| Texas Instruments Incorporated
| USB 3.0 TRANSCEIVER
| Marketing part#   Voltage Range   Package-type   Temperature
| TUSB1310IZAYR   2.97V - 3.465V   175 Ball NFBGA(175ZAY) -40C to 105C
| TUSB1310ZAY   2.97V - 3.465V   175 Ball NFBGA(175ZAY) -40C to 105C
| TUSB1310ZAYR   2.97V - 3.465V   175 Ball NFBGA(175ZAY) -40C to 105C
[IBIS Ver]   4.0
[File name]   tusb1310.ibs
[File Rev]   1.2
[Date]   05/06/2011
[Source]   Model built from TISPICE simulations at:
   Texas Instruments Incorporated.
   Analog-eLab, HPA
   12500 TI Blvd
   Dallas, TX -75243
   For Support e-mail: elab_scm_ibis@list.ti.com
[Notes]
   Rev 1.0: 06/04/2010
   - Initial version of model based on simulations from TISPICED
   - IBIS file covers only USB2.0 DP/DM and USB3.0 SSTXP/SSTXN pins only
   - For USB2.0, models are included for HS, FS and LS modes
   - For USB3.0, models are included for SATA1, SATA2 and No-De-Emphasis
   modes
   - Models are not matched to silicon or TISPICE.
   - Some of the POWER or GND balls are connected via the same net on
   package. Such ball names are commented out in the [Pin] section.
   For example, for pin B14, use the parastics of L12.
   - Warnings related to ccomp can be ignored. These reflect PVT conditions.
   Min ccomp corresponds PVT conditions related to Min. Max ccomp corresponds
   to PVT conditions related to Max
   - GND Clamp related warnings can be ignored as these reflect HS internal
   termination
   - Warnings related to USB2 LS pullup can be ignored as these are from
   simulations.
   Rev 1.1: 09/14/2010
   - Added model for DeEmphasis mode
   - Please use [Package Model] for system analysis
   - Removed parasitics from [Pin] for POWER and GND pins
   as they do not accurately represent pwr pkg parasitics
   [Package Model] includes mutuals and selfs more appropriately
   - C_comp although listed in numerical order of value are obtained from varying
   PVT conditions. For PVT conditions for each specific value refer the buffer
   description under respective [Model]. IBIS model user is responsible for using
   appropriate C_comp to simulate for Signal Integrity
   Where for TUSB1310,
   Nom PVT:  Nominal process, Typ Temperature, Typ Voltage
   Slow PVT: Weak process, Max Temperature, Min Voltage
   Fast PVT: Strong process, Min Temperatire, Max Voltage
   - ignore warning are related to usb3_WODE, please do not correct this error
   as IBIS parser does not correct IV-VT mismatch with single set of V-T
   waveforms.
   - non-monotonic arnings related to usb2_LS_RC and usb2_LS_R buffers are
   as they are seen in TISPICE simualations
   - [Driver Schedule] is interpreted differently by each system level simulator
   differently, if usual setup with it does not give appropriate results, please
   tie the MAIN and BOOST buffers as per buffer timing description under
   [Driver Schedule] keyword. For example, using HSPICE, refer DE_hspice.sp
   - Added USB High speed differential receiver model for SSRXP and SSRXN
   - Updated [Diff Pin] section.
   - Updated [Pin Mapping] section
   - Updated all USB2 model type to I/O and added Vinl and Vinh parameters
   - To test USB2 IBIS models using HSPICE look for spice set up files
   inside the TUSB1310 Correlation report
   Rev 1.2: 05/06/2011
   - [Driver Schedule] timing statements modified as per IBIS v5.0 spec.
   - Boost stage timing is set for a frequency of 1250MHz.
   - Depending on the speed grade( for various models, gen1/gen2/usb3.0 etc),
   user needs to alter the BOOST timing numbers for rise_off_dly and fall_off_dly
   usb3_de_BOOST   NA   0.2ns   NA   0.2ns
   This delay 0.2ns is valid for 1250MHz,(0.8ns period).
   Depending on the frequency, period divided by 4 needs to be used in
   DriverSchedule for BOOST
   -Ccomp interpretation needs to be assessed for accurate results. Ccomp that
   is assocaited with usb3_DE_MAIN is the complete number that includes ccomp for
   both BOOST and MAIN. Since MAIN buffer is on at all times and it is the boost
   that is turned on or ff, please set ccomp to suit your simulator's interpretation of
   IBIS v5.0 spec.
[Disclaimer] This product is designed as an aid for customers of Texas Instruments.
   No warranties, either expressed or implied, with respect to this third
   party software (if any) or with respect to its fitness for any
   particular purpose is claimed by Texas Instruments or the author. The
   software (if any) is provided solely on an "as is" basis. The entire
   risk as to its quality and performance is with the customer
[Copyright]   (C)Copyright 2010 Texas Instruments Incorporated.
   All rights reserved.
[Component]   TUSB1310
[Manufacturer]  Texas Instruments Incorporated
[Package]   |175-Ball NFBGA - ZAY package
|   typ   min   max
R_pkg   0.163   0.088   0.252
L_pkg   3.38E-09   1.90E-09   5.38E-09
C_pkg   8.14E-13   5.99E-13   1.14E-12
[Pin]   signal_name   model_name   R_pin   L_pin   C_pin
F12   AMUX   NC   0.123   2.67E-09   9.27E-13
|VSSA B13 B14 D12 E13 F13 G12 H13 J13 K12 L12 M12 M13 N13
B13   VSSA   GND
L12   VSSA   GND
B14   VSSA   GND
D12   VSSA   GND
E13   VSSA   GND
F13   VSSA   GND
G12   VSSA   GND
H13   VSSA   GND
J13   VSSA   GND
K12   VSSA   GND
M12   VSSA   GND
M13   VSSA   GND
N13   VSSA   GND
M14   CEXT   NC   0.206   4.22E-09   8.31E-13
A14   CEXTSS   NC   0.234   4.90E-09   1.14E-12
D10   CLKOUT   OC1840ETFZ   0.100   1.98E-09   8.20E-13
P13   DM   usb2   0.172   4.32E-09   1.07E-12
P14   DP   usb2   0.174   4.20E-09   1.07E-12
C9   ELAS_BUF_MODE   IC18THYPDFZ   0.107   2.15E-09   7.31E-13
G11   JTAG_TCK   IC18THYPUFZ   0.214   3.35E-09   1.03E-12
E11   JTAG_TDI   IC18THYPUFZ   0.189   3.25E-09   8.82E-13
F11   JTAG_TDO   OC1850BTFZ   0.111   2.08E-09   7.38E-13
D11   JTAG_TMS   IC18THYPUFZ   0.192   3.38E-09   8.24E-13
E12   JTAG_TRSTN   IC18THYPDFZ   0.125   2.65E-09   7.06E-13
L10   OUT_ENABLE   NC   0.112   2.43E-09   7.10E-13
A6   PCLK   OC1840ETFZ   0.171   3.49E-09   6.41E-13
J12   PHY_MODE0   IC18THYPUFZ   0.241   4.85E-09   9.10E-13
H12   PHY_MODE1   IC18THYPDFZ   0.142   3.44E-09   1.03E-12
J3   PHY_RESETN   IC18THYPUFZ   0.180   3.03E-09   7.47E-13
E3   PHY_STATUS   BC1850CTHYPDFZ   0.119   2.51E-09   8.98E-13
H3   POWER_DOWN0   IC18THY   0.117   2.62E-09   8.70E-13
G3   POWER_DOWN1   IC18THY   0.171   2.77E-09   7.44E-13
H11   PWRPRESENT   OC1850BTFZ   0.121   2.57E-09   1.13E-12
L14   R1EXT   NC   0.154   3.69E-09   8.94E-13
L13   R1EXTRTN   NC   0.147   3.48E-09   8.89E-13
L6   RATE   IC18THYPUFZ   0.165   2.42E-09   7.20E-13
C14   REFCLKN   PCIE_REFCLK   0.231   5.34E-09   1.03E-12
J4   REFCLKOUTN   OCML11G   0.114   2.10E-09   1.02E-12
K4   REFCLKOUTP   OCML11G   0.153   2.34E-09   9.10E-13
C13   REFCLKP   PCIE_REFCLK   0.227   4.61E-09   9.72E-13
J11   RESETN   IC18THYPUFZ   0.201   4.22E-09   9.66E-13
E2   RX_DATA0   OC1840ETFZ   0.130   2.81E-09   8.24E-13
D2   RX_DATA1   OC1840ETFZ   0.134   2.99E-09   7.99E-13
B4   RX_DATA10   OC1840ETFZ   0.199   4.05E-09   7.53E-13
B5   RX_DATA11   OC1840ETFZ   0.178   3.19E-09   8.95E-13
B8   RX_DATA12   OC1840ETFZ   0.152   2.79E-09   6.61E-13
A8   RX_DATA13   OC1840ETFZ   0.121   3.07E-09   7.16E-13
A9   RX_DATA14   OC1840ETFZ   0.170   3.44E-09   6.20E-13
B9   RX_DATA15   OC1840ETFZ   0.166   3.02E-09   7.47E-13
D1   RX_DATA2   OC1840ETFZ   0.227   4.32E-09   7.06E-13
C1   RX_DATA3   OC1840ETFZ   0.252   4.71E-09   8.47E-13
C2   RX_DATA4   OC1840ETFZ   0.163   3.81E-09   8.77E-13
B1   RX_DATA5   OC1840ETFZ   0.235   4.65E-09   8.12E-13
A2   RX_DATA6   OC1840ETFZ   0.169   3.85E-09   9.50E-13
A3   RX_DATA7   OC1840ETFZ   0.213   4.37E-09   7.74E-13
B3   RX_DATA8   OC1840ETFZ   0.145   3.78E-09   8.33E-13
A4   RX_DATA9   OC1840ETFZ   0.135   3.51E-09   7.98E-13
A7   RX_DATAK0   OC1840ETFZ   0.168   3.35E-09   6.79E-13
B7   RX_DATAK1   OC1840ETFZ   0.104   2.53E-09   6.88E-13
F3   RX_ELECIDLE   BC1850BTHYPDFZ   0.182   2.91E-09   6.62E-13
C8   RX_POLARITY   IC18THYPDFZ   0.088   1.90E-09   6.00E-13
C5   RX_STATUS0   OC1840ETFZ   0.165   2.80E-09   7.18E-13
C6   RX_STATUS1   OC1840ETFZ   0.106   2.38E-09   7.59E-13
C7   RX_STATUS2   OC1840ETFZ   0.153   2.66E-09   6.33E-13
D3   RX_TERMINATION  IC18THYPDFZ   0.196   2.85E-09   7.68E-13
F1   RX_VALID   OC1840ETFZ   0.137   3.33E-09   7.40E-13
F14   SSRXN   RXP_N   0.217   3.77E-09   8.52E-13
E14   SSRXP   RXP_N   0.218   3.97E-09   9.78E-13
J14   SSTXN   usb3_pcie   0.208   3.75E-09   8.55E-13
H14   SSTXP   usb3_pcie   0.208   3.69E-09   8.30E-13
D5   TMONITORN   NC   0.124   2.32E-09   7.64E-13
D6   TMONITORP   NC   0.144   2.12E-09   7.58E-13
K1   TX_CLK   IC18THY   0.139   3.72E-09   7.38E-13
P5   TX_DATA0   IC18THY   0.200   4.78E-09   1.04E-12
N4   TX_DATA1   IC18THY   0.228   3.82E-09   7.30E-13
L2   TX_DATA10   IC18THY   0.133   3.31E-09   9.07E-13
L3   TX_DATA11   IC18THY   0.201   4.08E-09   8.38E-13
J2   TX_DATA12   IC18THY   0.118   2.50E-09   7.09E-13
H1   TX_DATA13   IC18THY   0.134   3.42E-09   7.60E-13
H2   TX_DATA14   IC18THY   0.176   3.08E-09   6.61E-13
G2   TX_DATA15   IC18THY   0.176   3.06E-09   6.71E-13
P3   TX_DATA2   IC18THY   0.176   4.32E-09   9.73E-13
N3   TX_DATA3   IC18THY   0.161   3.67E-09   8.26E-13
P2   TX_DATA4   IC18THY   0.169   4.50E-09   9.20E-13
N2   TX_DATA5   IC18THY   0.223   4.47E-09   9.06E-13
P1   TX_DATA6   IC18THY   0.244   5.38E-09   9.19E-13
N1   TX_DATA7   IC18THY   0.165   4.33E-09   9.73E-13
M1   TX_DATA8   IC18THY   0.218   4.56E-09   8.63E-13
M2   TX_DATA9   IC18THY   0.154   4.25E-09   9.09E-13
J1   TX_DATAK0   IC18THY   0.207   4.34E-09   7.58E-13
G1   TX_DATAK1   IC18THY   0.131   3.15E-09   7.19E-13
L11   TX_DEEMPH0   IC18THYPUFZ   0.174   3.35E-09   9.12E-13
K11   TX_DEEMPH1   IC18THYPDFZ   0.135   3.43E-09   9.95E-13
M6   TX_DETRX_LPBK   IC18THYPDFZ   0.113   2.27E-09   6.84E-13
K3   TX_ELECIDLE   IC18THY   0.121   2.75E-09   7.86E-13
M9   TX_MARGIN0   IC18THYPDFZ   0.107   2.54E-09   6.97E-13
M10   TX_MARGIN1   IC18THYPDFZ   0.179   3.55E-09   7.60E-13
M11   TX_MARGIN2   IC18THYPDFZ   0.119   2.97E-09   8.34E-13
M4   TX_ONESZEROS   IC18THYPDFZ   0.193   3.05E-09   7.87E-13
M5   TX_SWING   IC18THYPDFZ   0.119   2.70E-09   7.42E-13
P11   ULPI_CLK   BC1850BTHYFZ   0.188   3.68E-09   7.74E-13
N9   ULPI_DATA0   BC1850BTHYPDFZ   0.171   3.57E-09   6.71E-13
P9   ULPI_DATA1   BC1850BTHYPDFZ   0.125   3.25E-09   7.44E-13
P8   ULPI_DATA2   BC1850BTHYPDFZ   0.125   3.30E-09   7.10E-13
N8   ULPI_DATA3   BC1850BTHYPDFZ   0.172   3.47E-09   6.86E-13
P7   ULPI_DATA4   BC1850BTHYPDFZ   0.170   3.49E-09   6.75E-13
N7   ULPI_DATA5   BC1850BTHYPDFZ   0.121   2.88E-09   5.99E-13
P6   ULPI_DATA6   BC1850BTHYPDFZ   0.127   3.10E-09   7.03E-13
N6   ULPI_DATA7   BC1850BTHYPDFZ   0.186   3.46E-09   7.64E-13
M7   ULPI_DIR   BC1850BTHYFZ   0.108   2.35E-09   6.35E-13
N11   ULPI_NXT   BC1850BTHYFZ   0.192   3.88E-09   7.83E-13
M8   ULPI_STP   BC1850BTHYPUFZ   0.105   2.23E-09   6.55E-13
N12   VBUS   POWER   0.146   3.56E-09   8.72E-13
|VDD1 A5 A10 B6 B10 E1 F2
B6   VDD1   POWER
A5   VDD1   POWER
A10   VDD1   POWER
B10   VDD1   POWER
E1   VDD1   POWER
F2   VDD1   POWER
|VDD2_VDD3 K2 L1 N5 P4
N5   VDD2_VDD3   POWER
K2   VDD2_VDD3   POWER
L1   VDD2_VDD3   POWER
P4   VDD2_VDD3   POWER
|VDD4 N10 P10
P10   VDD4   POWER
N10   VDD4   POWER
|VDD5 C11
C11   VDD5   POWER
|VDDA1P1SS D14 G13 K14
K14   VDDA1P1SS   POWER
D14   VDDA1P1SS   POWER
G13   VDDA1P1SS   POWER
|VDDA1P1SSPLL C12
C12   VDDA1P1SSPLL   POWER
|VDDA1P8USB2 N14
N14   VDDA1P8USB2   POWER
|VDDA3P3USB2 P12
P12   VDDA3P3USB2   POWER
|VDDD1P1SS D13 K13
D13   VDDD1P1SS   POWER
K13   VDDD1P1SS   POWER
|VDDR1P8SS A13
A13   VDDR1P8SS   POWER
|VDDS1 B2 C3 D4 D7 D8 D9 E4 F4
D8   VDDS1   POWER
B2   VDDS1   POWER
C3   VDDS1   POWER
D4   VDDS1   POWER
D7   VDDS1   POWER
D9   VDDS1   POWER
E4   VDDS1   POWER
F4   VDDS1   POWER
|VDDS2_VDDS3 G4 H4 L4 L5 M3
H4   VDDS2_VDDS3   POWER
G4   VDDS2_VDDS3   POWER
L4   VDDS2_VDDS3   POWER
L5   VDDS2_VDDS3   POWER
M3   VDDS2_VDDS3   POWER
|VDDS4 L7 L8 L9
L9   VDDS4   POWER
L7   VDDS4   POWER
L8   VDDS4   POWER
|VDDS5 C10
C10   VDDS5   POWER
|VPP C4
C4   VPP   POWER
|VSS1 F6 F7 F8 F9 G6 G7 G8 G9
F9   VSS1   GND
F6   VSS1   GND
F7   VSS1   GND
F8   VSS1   GND
G6   VSS1   GND
G7   VSS1   GND
G8   VSS1   GND
G9   VSS1   GND
|VSS2_VSS3 H6 H7 H8 J6 J7
H8   VSS2_VSS3   GND
H6   VSS2_VSS3   GND
H7   VSS2_VSS3   GND
J6   VSS2_VSS3   GND
J7   VSS2_VSS3   GND
|VSS4 H9 J8 J9
J8   VSS4   GND
H9   VSS4   GND
J9   VSS4   GND
|VSS5 B11
B11   VSS5   GND
|VSSOSC B12
B12   VSSOSC   GND
A12   XI   NC   0.155   3.66E-09   9.82E-13
A11   XO   NC   0.152   3.42E-09   8.35E-13
[Diff_pin]   inv_pin   vdiff   tdelay_typ   tdelay_min   tdelay_max
P14   P13   880mV   NA   NA   NA
|P14 and P13 are USB2 pins, 880mV is for HS, for LS/FS it is 7.2V
H14   J14   2200mV   NA   NA   NA
E14   F14   2200mV   NA   NA   NA
C13   C14   1450mV   NA   NA   NA
[Pin Mapping] pulldown_ref pullup_ref gnd_clamp_ref power_clamp_ref |ext_ref
F12 NC   NC | 1 BGA-F12 AMUX
L12 VSSABUS NC | 2 BGA-L12 VSSA
B13 VSSABUS NC
B14 VSSABUS NC
D12 VSSABUS NC
E13 VSSABUS NC
F13 VSSABUS NC
G12 VSSABUS NC
H13 VSSABUS NC
J13 VSSABUS NC
K12 VSSABUS NC
M12 VSSABUS NC
M13 VSSABUS NC
N13 VSSABUS NC
M14 NC   NC | 3 BGA-M14 CEXT
A14 NC   NC | 4 BGA-A14 CEXTSS
D10 NC   NC | 5 BGA-D10 CLKOUT
P13 VSSABUS VDDA3P3USB2BUS VSSABUS VDDA3P3USB2BUS| 6 BGA-P13 DM
P14 VSSABUS VDDA3P3USB2BUS VSSABUS VDDA3P3USB2BUS| 7 BGA-P14 DP
C9  NC NC | 8 BGA-C9 ELAS_BUF_MODE
G11 NC NC | 9 BGA-G11 JTAG_TCK
E11 NC NC | 10 BGA-E11 JTAG_TDI
F11 NC NC | 11 BGA-F11 JTAG_TDO
D11 NC NC | 12 BGA-D11 JTAG_TMS
E12 NC NC | 13 BGA-E12 JTAG_TRSTN
L10 NC NC | 14 BGA-L10 OUT_ENABLE
A6  NC NC | 15 BGA-A6 PCLK
J12 NC NC | 16 BGA-J12 PHY_MODE0
H12 NC NC | 17 BGA-H12 PHY_MODE1
J3  NC NC | 18 BGA-J3 PHY_RESETN
E3  NC NC | 19 BGA-E3 PHY_STATUS
H3  NC NC | 20 BGA-H3 POWER_DOWN0
G3  NC NC | 21 BGA-G3 POWER_DOWN1
H11 NC NC | 22 BGA-H11 PWRPRESENT
L14 NC NC | 23 BGA-L14 R1EXT
L13 NC NC  | 24 BGA-L13 R1EXTRTN
L6  NC NC | 25 BGA-L6 RATE
C14 VSS1BUS VDDD1P1SSBUS | 26 BGA-C14 REFCLKN
J4  NC NC | 27 BGA-J4 REFCLKOUTN
K4  NC NC | 28 BGA-K4 REFCLKOUTP
C13 VSS1BUS VDDD1P1SSBUS | 29 BGA-C13 REFCLKP
J11 NC NC | 30 BGA-J11 RESETN
E2  NC NC | 31 BGA-E2 RX_DATA0
D2  NC NC | 32 BGA-D2 RX_DATA1
B4  NC NC | 33 BGA-B4 RX_DATA10
B5  NC NC | 34 BGA-B5 RX_DATA11
B8  NC NC| 35 BGA-B8 RX_DATA12
A8  NC NC| 36 BGA-A8 RX_DATA13
A9  NC NC| 37 BGA-A9 RX_DATA14
B9  NC NC | 38 BGA-B9 RX_DATA15
D1  NC NC | 39 BGA-D1 RX_DATA2
C1  NC NC | 40 BGA-C1 RX_DATA3
C2  NC NC| 41 BGA-C2 RX_DATA4
B1  NC NC| 42 BGA-B1 RX_DATA5
A2  NC NC| 43 BGA-A2 RX_DATA6
A3  NC NC| 44 BGA-A3 RX_DATA7
B3  NC NC| 45 BGA-B3 RX_DATA8
A4  NC NC| 46 BGA-A4 RX_DATA9
A7  NC NC| 47 BGA-A7 RX_DATAK0
B7  NC NC| 48 BGA-B7 RX_DATAK1
F3  NC NC | 49 BGA-F3 RX_ELECIDLE
C8  NC NC | 50 BGA-C8 RX_POLARITY
C5  NC NC | 51 BGA-C5 RX_STATUS0
C6  NC NC | 52 BGA-C6 RX_STATUS1
C7  NC NC | 53 BGA-C7 RX_STATUS2
D3  NC NC| 54 BGA-D3 RX_TERMINATION
F1  NC NC| 55 BGA-F1 RX_VALID
F14 VSS1BUS VDDD1P1SSBUS| 56 BGA-F14 SSRXN
E14 VSS1BUS VDDD1P1SSBUS| 57 BGA-E14 SSRXP
J14 VSS1BUS VDDD1P1SSBUS VSS1BUS VDDD1P1SSBUS| 58 BGA-J14 SSTXN
H14 VSS1BUS VDDD1P1SSBUS VSS1BUS VDDD1P1SSBUS| 59 BGA-H14 SSTXP
D5  NC NC| 60 BGA-D5 TMONITORN
D6  NC NC| 61 BGA-D6 TMONITORP
K1  NC NC| 62 BGA-K1 TX_CLK
P5  NC NC| 63 BGA-P5 TX_DATA0
N4  NC NC| 64 BGA-N4 TX_DATA1
L2  NC NC| 65 BGA-L2 TX_DATA10
L3  NC NC| 66 BGA-L3 TX_DATA11
J2  NC NC| 67 BGA-J2 TX_DATA12
H1  NC NC| 68 BGA-H1 TX_DATA13
H2  NC NC| 69 BGA-H2 TX_DATA14
G2  NC NC| 70 BGA-G2 TX_DATA15
P3  NC NC| 71 BGA-P3 TX_DATA2
N3  NC NC| 72 BGA-N3 TX_DATA3
P2  NC NC| 73 BGA-P2 TX_DATA4
N2  NC NC| 74 BGA-N2 TX_DATA5
P1  NC NC| 75 BGA-P1 TX_DATA6
N1  NC NC| 76 BGA-N1 TX_DATA7
M1  NC NC| 77 BGA-M1 TX_DATA8
M2  NC NC| 78 BGA-M2 TX_DATA9
J1  NC NC| 79 BGA-J1 TX_DATAK0
G1  NC NC| 80 BGA-G1 TX_DATAK1
L11 NC NC| 81 BGA-L11 TX_DEEMPH0
K11 NC NC| 82 BGA-K11 TX_DEEMPH1
M6  NC NC| 83 BGA-M6 TX_DETRX_LPBK
K3  NC NC| 84 BGA-K3 TX_ELECIDLE
M9  NC NC| 85 BGA-M9 TX_MARGIN0
M10 NC NC| 86 BGA-M10 TX_MARGIN1
M11 NC NC| 87 BGA-M11 TX_MARGIN2
M4  NC NC| 88 BGA-M4 TX_ONESZEROS
M5  NC NC| 89 BGA-M5 TX_SWING
P11 NC NC| 90 BGA-P11 ULPI_CLK
N9  NC NC| 91 BGA-N9 ULPI_DATA0
P9  NC NC| 92 BGA-P9 ULPI_DATA1
P8  NC NC| 93 BGA-P8 ULPI_DATA2
N8  NC NC| 94 BGA-N8 ULPI_DATA3
P7  NC NC| 95 BGA-P7 ULPI_DATA4
N7  NC NC| 96 BGA-N7 ULPI_DATA5
P6  NC NC| 97 BGA-P6 ULPI_DATA6
N6  NC NC| 98 BGA-N6 ULPI_DATA7
M7  NC NC| 99 BGA-M7 ULPI_DIR
N11 NC NC| 100 BGA-N11 ULPI_NXT
M8  NC NC| 101 BGA-M8 ULPI_STP
N12 NC VBUSBUS| 102 BGA-N12 VBUS
B6  NC VDD1BUS| 103 BGA-B6 VDD1
A5  NC VDD1BUS
A10 NC VDD1BUS
B10 NC VDD1BUS
E1  NC VDD1BUS
F2  NC VDD1BUS
|VDD2_VDD3 K2 L1 N5 P4
N5  NC VDD2_3BUS
K2  NC VDD2_3BUS
L1  NC VDD2_3BUS
P4  NC VDD2_3BUS
|VDD4 N10 P10
P10 NC VDD4BUS
N10 NC VDD4BUS
|VDD5 C11
C11 NC VDD5BUS
|VDDA1P1SS D14 G13 K14
K14 NC VDDA1P1SSBUS
D14 NC VDDA1P1SSBUS
G13 NC VDDA1P1SSBUS
|VDDA1P1SSPLL C12
C12 NC VDDA1P1SSPLLBUS
|VDDA1P8USB2 N14
N14 NC VDDA1P8USB2BUS
|VDDA3P3USB2 P12
P12 NC VDDA3P3USB2BUS
|VDDD1P1SS D13 K13
D13 NC VDDD1P1SSBUS
K13 NC VDDD1P1SSBUS
|VDDR1P8SS A13
A13 NC VDDR1P8SSBUS
|VDDS1 B2 C3 D4 D7 D8 D9 E4 F4
D8  NC VDDS1BUS
B2  NC VDDS1BUS
C3  NC VDDS1BUS
D4  NC VDDS1BUS
D7  NC VDDS1BUS
D9  NC VDDS1BUS
E4  NC VDDS1BUS
F4  NC VDDS1BUS
|VDDS2_VDDS3 G4 H4 L4 L5 M3
H4  NC VDDS2_3BUS
G4  NC VDDS2_3BUS
L4  NC VDDS2_3BUS
L5  NC VDDS2_3BUS
M3  NC VDDS2_3BUS
|VDDS4 L7 L8 L9
L9  NC VDDS4BUS
L7  NC VDDS4BUS
L8  NC VDDS4BUS
|VDDS5 C10
C10 NC VDDS5BUS
|VPP C4
C4  NC VPPBUS
|VSS1 F6 F7 F8 F9 G6 G7 G8 G9
F9  VSS1BUS NC
F6  VSS1BUS NC
F7  VSS1BUS NC
F8  VSS1BUS NC
G6  VSS1BUS NC
G7  VSS1BUS NC
G8  VSS1BUS NC
G9  VSS1BUS NC
|VSS2_VSS3 H6 H7 H8 J6 J7
H8  VSS2_3BUS NC
H6  VSS2_3BUS NC
H7  VSS2_3BUS NC
J6  VSS2_3BUS NC
J7  VSS2_3BUS NC
|VSS4 H9 J8 J9
J8  VSS4BUS NC
H9  VSS4BUS NC
J9  VSS4BUS NC
|VSS5 B11
B11 VSS5BUS NC
|VSSOSC B12
B12 VSSOSC NC
A12 NC NC| 123 BGA-A12 XI
A11 NC NC| 124 BGA-A11 XO
[Model Selector] usb2
usb2_HS_R   USB 2.0 High Speed mode, for DP/DM pin 240MHz
usb2_HS_RC   USB 2.0 High Speed mode, for DP/DM pin 240MHz, with Cfixture
usb2_FS_R   USB 2.0 Fast Speed mode, for DP/DM pin 6MHz
usb2_FS_RC   USB 2.0 Fast Speed mode, for DP/DM pin 6MHz, with Cfixture
usb2_LS_RC   USB 2.0 Low  Speed mode, for DP/DM pin 750kHz, with Cfixture
usb2_LS_R   USB 2.0 Low  Speed mode, for DP/DM pin 750kHz
[Model Selector] usb3_pcie
usb3_DE   USB 3.0 De-Emphasis mode, best at 1.25GHz
usb3_WODE   USB 3.0 No De-Emphasis mode, for SSTXP/N 2.5GHz
usb3_SATA1   USB 3.0 SATA1 mode, for SSTXP/N 750MHz
usb3_SATA2   USB 3.0 SATA2 mode, for SSTXP/N 1.5GHz
pcie_GEN2   PCI-E 2.5GHz  GEN2 model
pcie_GEN1   PCI-E 1.25GHz GEN1 model
|   175 Ball nFBGA ZAY package
[Define Package Model]  TUSB1310ZAY_PakSiE_020410
[Manufacturer]   Texas Instruments, Inc
[OEM]   Texas Instruments, Inc
[Description]   175-Ball nFBGA
[Number Of Pins]   124
[Pin Numbers]
F12 | 1 BGA-F12 AMUX
L12 | 2 BGA-L12 VSSA
M14 | 3 BGA-M14 CEXT
A14 | 4 BGA-A14 CEXTSS
D10 | 5 BGA-D10 CLKOUT
P13 | 6 BGA-P13 DM
P14 | 7 BGA-P14 DP
C9 | 8 BGA-C9 ELAS_BUF_MODE
G11 | 9 BGA-G11 JTAG_TCK
E11 | 10 BGA-E11 JTAG_TDI
F11 | 11 BGA-F11 JTAG_TDO
D11 | 12 BGA-D11 JTAG_TMS
E12 | 13 BGA-E12 JTAG_TRSTN
L10 | 14 BGA-L10 OUT_ENABLE
A6 | 15 BGA-A6 PCLK
J12 | 16 BGA-J12 PHY_MODE0
H12 | 17 BGA-H12 PHY_MODE1
J3 | 18 BGA-J3 PHY_RESETN
E3 | 19 BGA-E3 PHY_STATUS
H3 | 20 BGA-H3 POWER_DOWN0
G3 | 21 BGA-G3 POWER_DOWN1
H11 | 22 BGA-H11 PWRPRESENT
L14 | 23 BGA-L14 R1EXT
L13 | 24 BGA-L13 R1EXTRTN
L6 | 25 BGA-L6 RATE
C14 | 26 BGA-C14 REFCLKN
J4 | 27 BGA-J4 REFCLKOUTN
K4 | 28 BGA-K4 REFCLKOUTP
C13 | 29 BGA-C13 REFCLKP
J11 | 30 BGA-J11 RESETN
E2 | 31 BGA-E2 RX_DATA0
D2 | 32 BGA-D2 RX_DATA1
B4 | 33 BGA-B4 RX_DATA10
B5 | 34 BGA-B5 RX_DATA11
B8 | 35 BGA-B8 RX_DATA12
A8 | 36 BGA-A8 RX_DATA13
A9 | 37 BGA-A9 RX_DATA14
B9 | 38 BGA-B9 RX_DATA15
D1 | 39 BGA-D1 RX_DATA2
C1 | 40 BGA-C1 RX_DATA3
C2 | 41 BGA-C2 RX_DATA4
B1 | 42 BGA-B1 RX_DATA5
A2 | 43 BGA-A2 RX_DATA6
A3 | 44 BGA-A3 RX_DATA7
B3 | 45 BGA-B3 RX_DATA8
A4 | 46 BGA-A4 RX_DATA9
A7 | 47 BGA-A7 RX_DATAK0
B7 | 48 BGA-B7 RX_DATAK1
F3 | 49 BGA-F3 RX_ELECIDLE
C8 | 50 BGA-C8 RX_POLARITY
C5 | 51 BGA-C5 RX_STATUS0
C6 | 52 BGA-C6 RX_STATUS1
C7 | 53 BGA-C7 RX_STATUS2
D3 | 54 BGA-D3 RX_TERMINATION
F1 | 55 BGA-F1 RX_VALID
F14 | 56 BGA-F14 SSRXN
E14 | 57 BGA-E14 SSRXP
J14 | 58 BGA-J14 SSTXN
H14 | 59 BGA-H14 SSTXP
D5 | 60 BGA-D5 TMONITORN
D6 | 61 BGA-D6 TMONITORP
K1 | 62 BGA-K1 TX_CLK
P5 | 63 BGA-P5 TX_DATA0
N4 | 64 BGA-N4 TX_DATA1
L2 | 65 BGA-L2 TX_DATA10
L3 | 66 BGA-L3 TX_DATA11
J2 | 67 BGA-J2 TX_DATA12
H1 | 68 BGA-H1 TX_DATA13
H2 | 69 BGA-H2 TX_DATA14
G2 | 70 BGA-G2 TX_DATA15
P3 | 71 BGA-P3 TX_DATA2
N3 | 72 BGA-N3 TX_DATA3
P2 | 73 BGA-P2 TX_DATA4
N2 | 74 BGA-N2 TX_DATA5
P1 | 75 BGA-P1 TX_DATA6
N1 | 76 BGA-N1 TX_DATA7
M1 | 77 BGA-M1 TX_DATA8
M2 | 78 BGA-M2 TX_DATA9
J1 | 79 BGA-J1 TX_DATAK0
G1 | 80 BGA-G1 TX_DATAK1
L11 | 81 BGA-L11 TX_DEEMPH0
K11 | 82 BGA-K11 TX_DEEMPH1
M6 | 83 BGA-M6 TX_DETRX_LPBK
K3 | 84 BGA-K3 TX_ELECIDLE
M9 | 85 BGA-M9 TX_MARGIN0
M10 | 86 BGA-M10 TX_MARGIN1
M11 | 87 BGA-M11 TX_MARGIN2
M4 | 88 BGA-M4 TX_ONESZEROS
M5 | 89 BGA-M5 TX_SWING
P11 | 90 BGA-P11 ULPI_CLK
N9 | 91 BGA-N9 ULPI_DATA0
P9 | 92 BGA-P9 ULPI_DATA1
P8 | 93 BGA-P8 ULPI_DATA2
N8 | 94 BGA-N8 ULPI_DATA3
P7 | 95 BGA-P7 ULPI_DATA4
N7 | 96 BGA-N7 ULPI_DATA5
P6 | 97 BGA-P6 ULPI_DATA6
N6 | 98 BGA-N6 ULPI_DATA7
M7 | 99 BGA-M7 ULPI_DIR
N11 | 100 BGA-N11 ULPI_NXT
M8 | 101 BGA-M8 ULPI_STP
N12 | 102 BGA-N12 VBUS
B6 | 103 BGA-B6 VDD1
N5 | 104 BGA-N5 VDD2_VDD3
P10 | 105 BGA-P10 VDD4
C11 | 106 BGA-C11 VDD5
K14 | 107 BGA-K14 VDDA1P1SS
C12 | 108 BGA-C12 VDDA1P1SSPLL
N14 | 109 BGA-N14 VDDA1P8USB2
P12 | 110 BGA-P12 VDDA3P3USB2
D13 | 111 BGA-D13 VDDD1P1SS
A13 | 112 BGA-A13 VDDR1P8SS
D8 | 113 BGA-D8 VDDS1
H4 | 114 BGA-H4 VDDS2_VDDS3
L9 | 115 BGA-L9 VDDS4
C10 | 116 BGA-C10 VDDS5
C4 | 117 BGA-C4 VPP
F9 | 118 BGA-F9 VSS1
H8 | 119 BGA-H8 VSS2_VSS3
J8 | 120 BGA-J8 VSS4
B11 | 121 BGA-B11 VSS5
B12 | 122 BGA-B12 VSSOSC
A12 | 123 BGA-A12 XI
A11 | 124 BGA-A11 XO
[Model Data]
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[End Model Data]
[End Package Model]
|USB 3.0 De-Emphasis mode, for SSTXP/SSTXN pins 2.5Gbps(1.25GHz to De-Emphasis)
[Model]   usb3_DE
Model_type   Output
Vmeas = 1.1
Vref = 1.1
Rref = 50
|   typ   min   max
|   (TYP PVT)   (Fast PVT) (Slow PVT)
C_comp   0.5286pF   0.5195pF   0.5464pF
[Driver Schedule]
| Model_name   Rise_on_dly Rise_off_dly Fall_on_dly Fall_off_dly
usb3_de_MAIN   0.0   NA   0.0   NA
usb3_de_BOOST   NA   0.2ns   NA   0.2ns
[Voltage Range]   1.1   0.99   1.155
[Temperature Range]   27   105   -40
[Pullup Reference]   1.1   0.99   1.155
[Pulldown Reference]   0   0   0
[Power Clamp Reference]   1.1   0.99   1.155
[GND Clamp Reference]   0   0   0
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[Ramp]
R_load = 50
|   typ   min   max
dV/dt_r   0.972315/1.549e-011   0.988218/1.8606e-011   0.957162/1.40763e-011
dV/dt_f   0.972312/7.7916e-012   0.988183/1.21282e-011  0.957081/6.00194e-012
|PCIE GEN2 De-Emphasis mode, for SSTXP/SSTXN pins 5Gbps(2.5GHz to De-Emphasis)
[Model]   pcie_GEN2
Model_type   Output
Vmeas = 1.1
Vref = 1.1
Rref = 50
|   typ   min   max
|   (TYP PVT)   (Fast PVT) (Slow PVT)
C_comp   0.5286pF   0.5195pF   0.5464pF
[Driver Schedule]
| Model_name   Rise_on_dly Rise_off_dly Fall_on_dly Fall_off_dly
usb3_de_MAIN   0.0nS   NA   0.0ns   NA
usb3_de_BOOST   NA   0.2nS   NA   0.2nS
[Voltage Range]   1.1   0.99   1.155
[Temperature Range]   27   105   -40
[Pullup Reference]   1.1   0.99   1.155
[Pulldown Reference]   0   0   0
[Power Clamp Reference]   1.1   0.99   1.155
[GND Clamp Reference]   0   0   0
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[Ramp]
R_load = 50
|   typ   min   max
dV/dt_r   0.972315/1.549e-011   0.988218/1.8606e-011   0.957162/1.40763e-011
dV/dt_f   0.972312/7.7916e-012   0.988183/1.21282e-011  0.957081/6.00194e-012
|PCIE GEN1 De-Emphasis mode, for SSTXP/SSTXN pins 2.5Gbps(1.25GHz to De-Emphasis)
[Model]   pcie_GEN1
Model_type   Output
Vmeas = 1.1
Vref = 1.1
Rref = 50
|   typ   min   max
|   (TYP PVT)   (Fast PVT) (Slow PVT)
C_comp   0.5286pF   0.5195pF   0.5464pF
[Driver Schedule]
| Model_name   Rise_on_dly Rise_off_dly Fall_on_dly Fall_off_dly
usb3_de_MAIN   0.0nS   NA   0.0ns   NA
usb3_de_BOOST   NA   0.4nS   NA   0.4nS
[Voltage Range]   1.1   0.99   1.155
[Temperature Range]   27   105   -40
[Pullup Reference]   1.1   0.99   1.155
[Pulldown Reference]   0   0   0
[Power Clamp Reference]   1.1   0.99   1.155
[GND Clamp Reference]   0   0   0
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[Ramp]
R_load = 50
|   typ   min   max
dV/dt_r   0.972315/1.549e-011   0.988218/1.8606e-011   0.957162/1.40763e-011
dV/dt_f   0.972312/7.7916e-012   0.988183/1.21282e-011  0.957081/6.00194e-012
| Models and submodels in the file (26): RXP_N (Input), PCIE_REFCLK (Input), usb2_FS_R (I/O), usb2_FS_RC (I/O), usb2_HS_R (I/O), usb2_HS_RC (I/O), usb2_LS_R (I/O), usb2_LS_RC (I/O), usb3_WODE (Output), usb3_SATA1 (Output), usb3_SATA2 (Output), usb3_DE (Output), usb3_de_MAIN (Output), usb3_de_BOOST (Open_drain), pcie_GEN2 (Output), pcie_GEN1 (Output), IC18THY (Input), IC18THYPDFZ (Input), IC18THYPUFZ (Input), OC1840ETFZ (3-state), OC1850BTFZ (3-state), OCML11G (Output), BC1850BTHYFZ (I/O), BC1850BTHYPDFZ (I/O), BC1850CTHYPDFZ (I/O), BC1850BTHYPUFZ (I/O)
